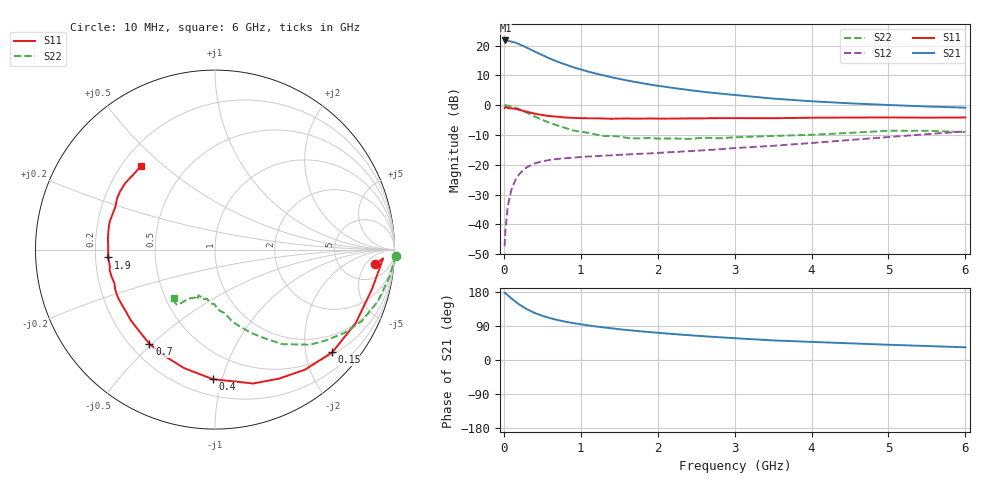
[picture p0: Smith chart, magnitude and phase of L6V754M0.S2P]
!  INFINEON TECHNOLOGIES Small Signal Semiconductors
! BFR380L3 , Si-NPN RF-Transistor in TSLP-3-1
!  Vce=0.75 V,  Ic=4 mA
! Common Emitter S-Parameters:  07. March 2005
#  GHz  S  MA  R  50
! f  S11  S21  S12  S22
! GHz  Mag  Ang  Mag  Ang  Mag  Ang  Mag  Ang
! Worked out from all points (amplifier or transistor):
!   36 points, 10 MHz to 6 GHz, reference 50 ohm
!   highest |S21| = 21.7 dB at 20 MHz (marker M1)
!   |S21| within 3 dB of that: start of sweep to 343.9 MHz
!   unconditionally stable (mu >= 1): 2.351 GHz to 4.939 GHz
!   at 250 MHz: K = 0.15, MSG = 20.9 dB, |S12| = -21.8 dB
!   at 1.4 GHz: K = 0.73, MSG = 13.1 dB, |S12| = -16.8 dB
!   at 6 GHz: K = 0.97, MSG = 4.0 dB, |S12| = -8.8 dB
!   S11 on the Smith chart (normalised r, x): 10 MHz: 11, -9; 150 MHz: 0.55, -2.56; 400 MHz: 0.31, -0.93; 700 MHz: 0.28, -0.49; 1.9 GHz: 0.25, -0.03; 6 GHz: 0.28, +0.42
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0.01  0.8962 -5.2  12.15 176.6  0.0043 88.1  1.01 -1.9
0.02  0.9383 -3.0  12.2 176.7  0.0075 92.0  1 -3.8
0.05  0.9018 -14.2  12.04 171.1  0.0199 84.3  0.9833 -9.0
0.1  0.8845 -27.5  11.67 162.5  0.0384 76.0  0.9518 -17.6
0.15  0.8687 -41.2  11.21 154.2  0.0554 68.3  0.9104 -25.9
0.2  0.8361 -53.1  10.56 146.6  0.0694 63.3  0.859 -32.6
0.25  0.8026 -63.6  9.894 140.2  0.081 57.5  0.7988 -39.3
0.3  0.7756 -74.1  9.195 134.0  0.091 53.5  0.7493 -45.0
0.4  0.7219 -91.0  7.975 124.2  0.1053 46.5  0.6461 -54.6
0.5  0.6825 -104.5  6.924 116.7  0.1143 42.4  0.5661 -60.8
0.6  0.6551 -115.9  6.045 110.4  0.1206 39.1  0.5046 -66.7
0.7  0.6397 -124.8  5.369 105.5  0.1254 37.3  0.4548 -71.5
0.9  0.6125 -139.9  4.344 97.4  0.1311 35.2  0.3771 -79.4
1.1  0.6028 -149.8  3.653 91.1  0.1376 34.9  0.3436 -85.2
1.4  0.5907 -161.6  2.937 83.7  0.1441 35.3  0.3043 -91.9
1.9  0.5985 -175.8  2.22 73.6  0.155 38.8  0.2825 -102.9
2.2  0.5956 177.8  1.948 68.5  0.1636 41.3  0.2765 -104.9
2.8  0.6062 167.0  1.571 60.1  0.1816 46.5  0.2785 -113.0
3.5  0.6039 156.9  1.29 51.7  0.2081 50.3  0.3048 -117.1
4.5  0.6203 148.3  1.074 44.0  0.2606 55.5  0.3427 -121.5
5.5  0.6177 137.9  0.951 36.9  0.3261 56.3  0.3718 -126.6
6  0.6218 131.8  0.908 33.5  0.3633 55.5  0.3523 -130.7
